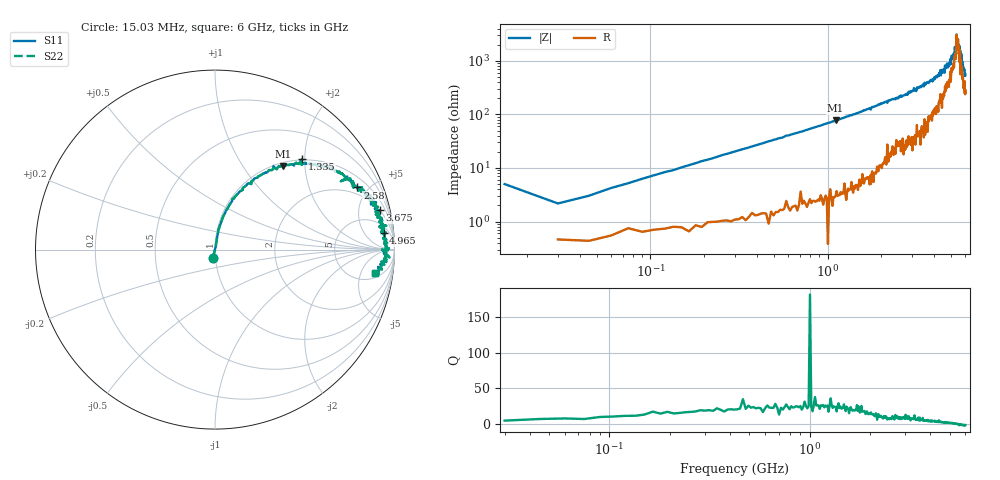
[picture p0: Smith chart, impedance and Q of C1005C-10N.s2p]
!	Network	Analyzer	HP8753E.07.74:	Oct	30	2002	Serial	No.	JP38451487
!	Hewlett-Packard
!	7	Sep	2009	8:37:45
!	Frequency	S11	S21	S12	S22
#	HZ	S	RI	R	50
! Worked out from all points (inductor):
!   400 points, 15.03 MHz to 6 GHz, reference 50 ohm
!   read as one part in series: L = 10.9 nH near 45.03 MHz
!   highest Q = 26.1 at 1.11 GHz (marker M1), where L = 11.1 nH
!   self-resonance near 5.438 GHz
!   S11 on the Smith chart (normalised r, x): 15.03 MHz: 0.97, -0.10; 1.335 GHz: 0.98, +1.94; 2.58 GHz: 1.55, +4.26; 3.675 GHz: 1.95, +8.01; 4.965 GHz: 9, +15; 6 GHz: 7, -9
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1.502992e7  -0.0128 -0.0495  1.01 0.0495  1.01 0.0495  -0.0128 -0.0495
3.002985e7  0.00513 0.0211  0.995 -0.0211  0.995 -0.0211  0.00513 0.0211
1.200294e8  0.0141 0.0815  0.986 -0.0815  0.986 -0.0815  0.0141 0.0815
2.850286e8  0.0451 0.183  0.955 -0.183  0.955 -0.183  0.0451 0.183
1.020025e9  0.336 0.452  0.664 -0.452  0.664 -0.452  0.336 0.452
1.110024e9  0.378 0.466  0.622 -0.466  0.622 -0.466  0.378 0.466
1.335023e9  0.485 0.505  0.515 -0.505  0.515 -0.505  0.485 0.505
2.01002e9  0.701 0.423  0.299 -0.423  0.299 -0.423  0.701 0.423
2.580017e9  0.793 0.346  0.207 -0.346  0.207 -0.346  0.793 0.346
3.015015e9  0.866 0.304  0.134 -0.304  0.134 -0.304  0.866 0.304
3.675012e9  0.919 0.22  0.081 -0.22  0.081 -0.22  0.919 0.22
4.00501e9  0.926 0.175  0.0739 -0.175  0.0739 -0.175  0.926 0.175
4.965005e9  0.939 0.0908  0.0611 -0.0908  0.0611 -0.0908  0.939 0.0908
5.010005e9  0.944 0.068  0.0555 -0.068  0.0555 -0.068  0.944 0.068
5.325003e9  0.948 0.0303  0.0517 -0.0303  0.0517 -0.0303  0.948 0.0303
5.355003e9  0.969 0.0054  0.0306 -0.0054  0.0306 -0.0054  0.969 0.0054
5.370003e9  0.952 0.0154  0.0482 -0.0154  0.0482 -0.0154  0.952 0.0154
5.445003e9  0.963 -0.00388  0.0373 0.00388  0.0373 0.00388  0.963 -0.00388
5.535002e9  0.931 0.00107  0.0694 -0.00107  0.0694 -0.00107  0.931 0.00107
5.565002e9  0.972 -0.0434  0.0278 0.0434  0.0278 0.0434  0.972 -0.0434
5.625002e9  0.954 -0.0695  0.0458 0.0695  0.0458 0.0695  0.954 -0.0695
6e9  0.894 -0.13  0.106 0.13  0.106 0.13  0.894 -0.13
